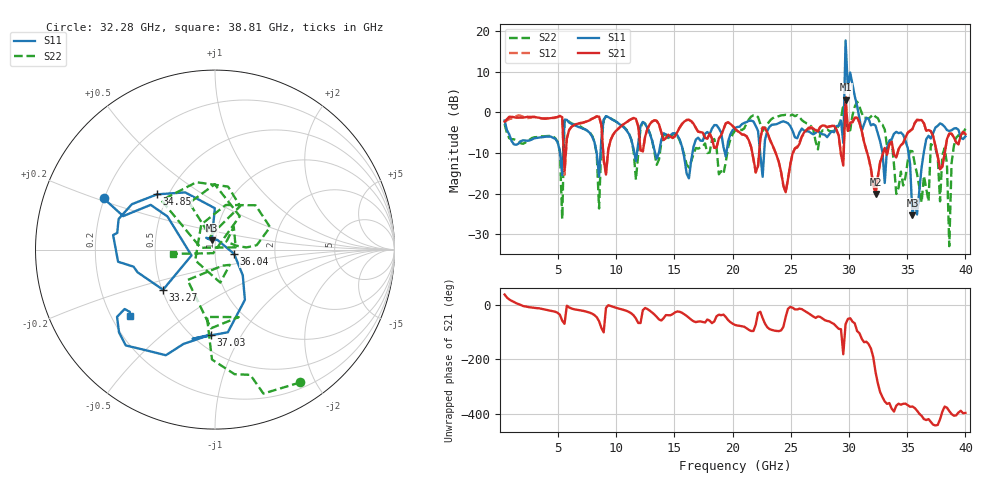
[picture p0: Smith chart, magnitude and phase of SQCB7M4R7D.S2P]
! Network Analyzer HP8722ES.07.66: Jul 25, 2000 Serial No. US39175408
! 26 Oct 2004  14:24:06
! Frequency  S11  S21  S12  S22
# HZ  S  DB R  50
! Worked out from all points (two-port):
!   201 points, 400 MHz to 40 GHz, reference 50 ohm
!   highest |S21| = 3.08 dB at 29.7 GHz (marker M1); lowest = -20.1 dB at 32.28 GHz (marker M2)
!   |S21| within 3 dB of the highest: 29.66735 GHz to 29.78147 GHz (114.1 MHz wide, 0.384 % of centre)
!   lowest |S11| = -25.3 dB at 35.45 GHz (marker M3), VSWR 1.11, Z = 48 + j4.9 ohm
!   |S11| at or under -10 dB: 8.308 GHz to 8.643 GHz (335.6 MHz wide, 3.96 % of centre); 15.76 GHz to 16.54 GHz (786.2 MHz wide, 4.87 % of centre); 35.11 GHz to 36.42 GHz (1.315 GHz wide, 3.68 % of centre)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
!   |S22| runs from -32.9 to 2.6 dB; largest |S21 - S12| = 0.7
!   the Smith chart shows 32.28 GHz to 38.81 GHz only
!   S11 on the Smith chart (normalised r, x): 32.28 GHz: 0.20, +0.21; 33.27 GHz: 0.51, -0.26; 34.85 GHz: 0.43, +0.33; 36.04 GHz: 1.24, -0.06; 37.03 GHz: 0.61, -0.74; 38.81 GHz: 0.28, -0.32
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4e8  -2.05 -53.9  -2.31 37.5  -2.44 42.5  -2.92 -46.1
5.35e9  -15.53 -47.2  -1.21 -58.3  -1.20 -59.3  -26.27 -41.0
7.132e9  -4.07 -102.1  -2.54 -22.2  -2.60 -22.9  -3.94 -122.5
1.3666e10  -9.92 -38.1  -2.98 -53.6  -3.05 -53.7  -11.62 -59.6
2.02e10  -3.88 -0.3  -4.04 -73.9  -3.99 -73.1  -4.52 7.4
2.6932e10  -5.43 119.7  -4.02 -43.3  -3.60 -43.9  -4.30 -34.6
2.9506e10  -7.56 11.6  -13.13 178.3  -11.56 -132.5  1.85 29.3
2.9704e10  17.65 -35.3  3.08 -71.0  3.80 -44.4  -1.85 -66.8
2.9902e10  5.55 -80.7  -4.59 -51.9  -4.58 -51.1  -4.50 10.1
3.01e10  9.76 -105.9  -2.61 -49.4  -2.63 -49.5  -4.43 22.7
3.0298e10  6.85 -139.0  -2.49 -61.7  -2.29 -61.3  -0.77 16.7
3.0496e10  3.89 -147.1  -1.38 -68.2  -1.36 -67.3  1.41 1.1
3.0694e10  1.57 3.4  -1.33 -96.7  -1.30 -96.0  2.59 158.0
3.2278e10  -3.31 155.3  -20.11 113.1  -20.02 110.5  -1.12 -57.3
3.3268e10  -8.74 -142.3  -10.46 -3.6  -10.21 -3.5  -8.45 -96.8
3.3466e10  -6.94 -163.7  -7.86 -0.5  -7.82 -0.8  -7.99 -70.7
3.4852e10  -7.02 136.3  -6.20 -2.8  -6.06 -1.9  -15.95 118.7
3.5446e10  -25.34 109.6  -4.17 -13.2  -4.08 -12.7  -9.59 22.2
3.604e10  -19.24 -12.6  -1.94 -39.7  -1.94 -38.9  -18.40 10.5
3.703e10  -6.48 -92.8  -4.67 -69.9  -4.67 -68.8  -7.85 137.4
3.8812e10  -4.44 -141.8  -5.28 -40.9  -5.27 -40.7  -12.52 -174.2
4e10  -5.93 -141.4  -5.41 -36.9  -5.35 -35.4  -4.04 125.9
